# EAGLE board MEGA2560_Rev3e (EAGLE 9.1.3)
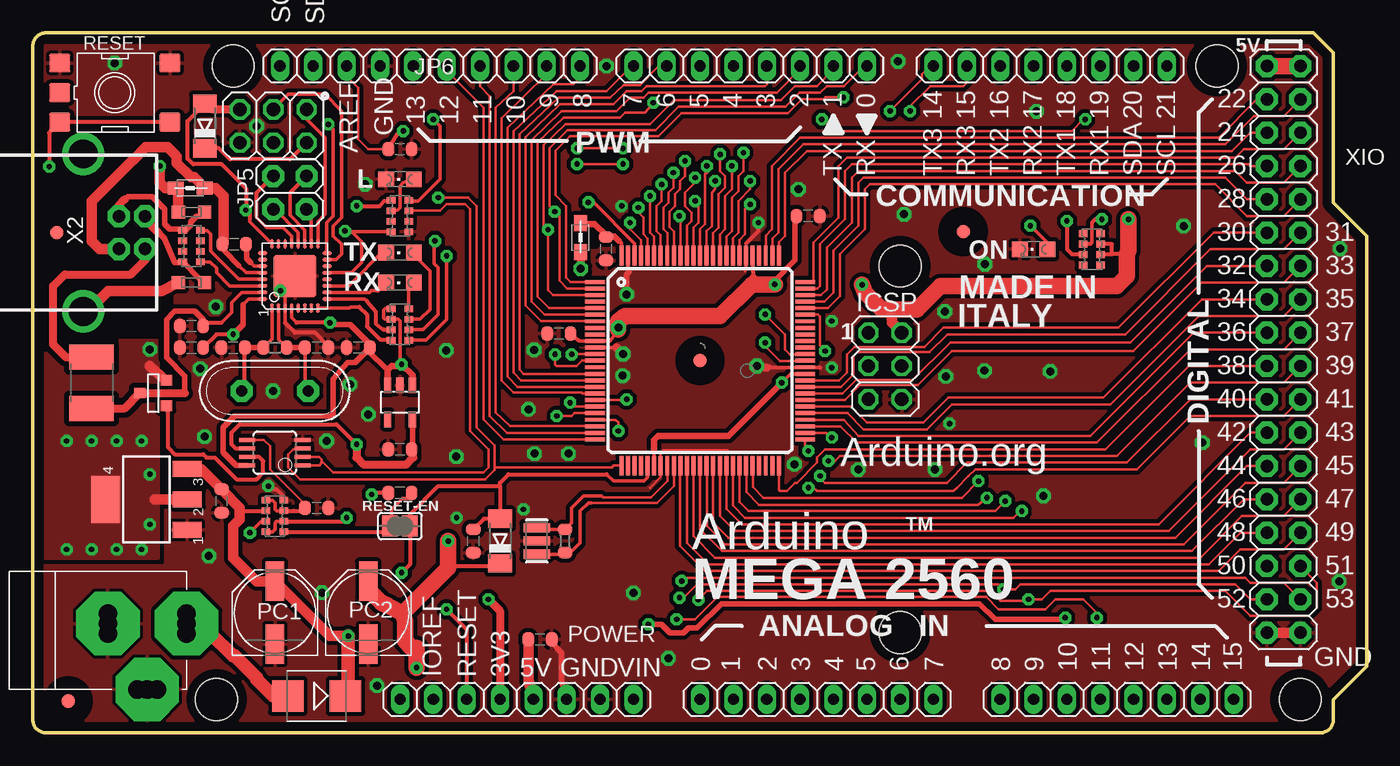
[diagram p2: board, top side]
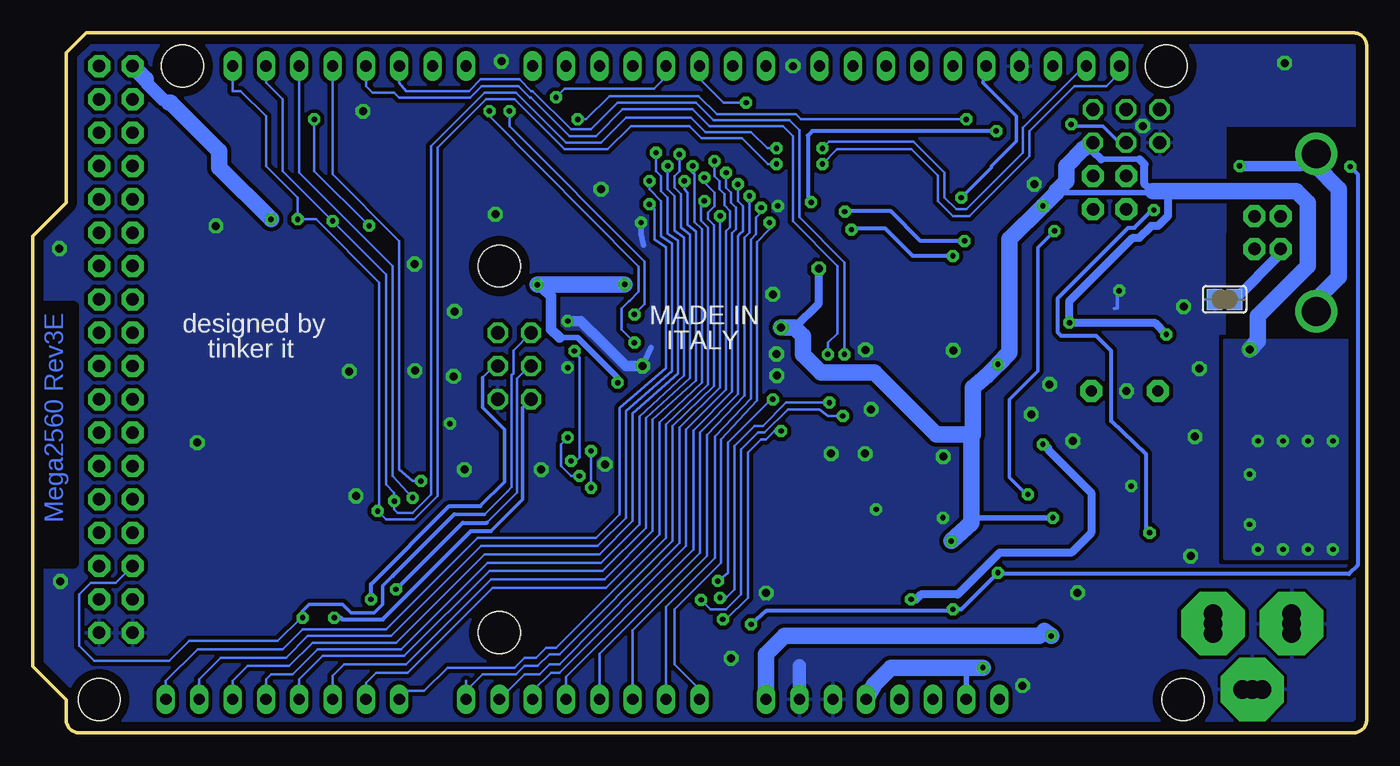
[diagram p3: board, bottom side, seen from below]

Size 101.6 x 53.34 mm. Coordinates in mm from the lower left corner, seen from the top.
Outline: 97.54,53.34 99.06,51.82 99.06,40.39 101.6,37.85 101.6,5.08 99.06,2.54 99.06,1 arc-90 98.06,0 1,0 arc-90 0,1 0,52.34 arc-90 1,53.34 97.54,53.34
Copper layers (1*16): Top 0.035mm / dielectric 1.5mm / Bottom 0.035mm
Design rules "ArduinoMega *": minimum track width 8mil, minimum drill 16mil, track to track 7mil, track to pad 7mil, pad to pad 8mil, via to via 10mil, smd to smd 7mil, copper to edge 27mil, drill to drill 12mil, minimum pad ring 10mil, minimum via ring 10mil, stop-mask expansion 2mil, vias tented up to drill 24mil, thermal gap 10mil
Net classes: 0 default: width 0.203 mm, drill 0.406 mm, clearance 0.203 mm; 1 power: width 0.61 mm, drill 0.406 mm, clearance 0.203 mm; 2 gnd: width 0.305 mm, drill 0.406 mm, clearance 0.203 mm; 3 power usb: width 0.508 mm, drill 0.406 mm, clearance 0.203 mm
Holes 3.2 mm at 96.55,2.55 15.27,50.81 90.2,50.81 14,2.55 66.07,35.57 66.07,7.63
tRestrict: area 42.5,37.2 to 42.9,37.4
bRestrict: 3 lines

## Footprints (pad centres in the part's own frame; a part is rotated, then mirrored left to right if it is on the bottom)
1X08 = drill 0.85 pad 1.422 long: 1 -8.89,0; 2 -6.35,0; 3 -3.81,0; 4 -1.27,0; 5 1.27,0; 6 3.81,0; 7 6.35,0; 8 8.89,0
C0603-ROUND = smd 0.898 x 1.1: 1 -0.889,0; 2 0.889,0
SMB = smd 2.4 x 2.4: A 2.2,0; C -2.2,0
MINIMELF = smd 1.4 x 1.8: A 1.7,0; C -1.7,0
L1812 = smd 1.9 x 3.4: 1 -1.95,0; 2 1.95,0
FIDUCIA-MOUNT = smd 1.016 x 1.016: P$1 0,0
SJ = smd 1.168 x 1.6: 1 -0.762,0; 2 0.762,0
LINEAR_SOT223 = smd 1.219 x 2.235: 1 -2.311,-3.099; 2 0,-3.099; 3 2.311,-3.099 | smd 3.6 x 2.2: 4 0,3.099
TQFP100 = smd 1.5 x 0.3: 1 -8,6; 2 -8,5.5; 3 -8,5; 4 -8,4.5; 5 -8,4; 6 -8,3.5; 7 -8,3; 8 -8,2.5; 9 -8,2; 10 -8,1.5; 11 -8,1; 12 -8,0.5; 13 -8,0; 14 -8,-0.5; 15 -8,-1; 16 -8,-1.5; 17 -8,-2; 18 -8,-2.5; 19 -8,-3; 20 -8,-3.5; 21 -8,-4; 22 -8,-4.5; 23 -8,-5; 24 -8,-5.5; 25 -8,-6; 51 8,-6; 52 8,-5.5; 53 8,-5; 54 8,-4.5; 55 8,-4; 56 8,-3.5; 57 8,-3; 58 8,-2.5; 59 8,-2; 60 8,-1.5; 61 8,-1; 62 8,-0.5; 63 8,0; 64 8,0.5; 65 8,1; 66 8,1.5; 67 8,2; 68 8,2.5; 69 8,3; 70 8,3.5; 71 8,4; 72 8,4.5; 73 8,5; 74 8,5.5; 75 8,6 | smd 0.3 x 1.5: 26 -6,-8; 27 -5.5,-8; 28 -5,-8; 29 -4.5,-8; 30 -4,-8; 31 -3.5,-8; 32 -3,-8; 33 -2.5,-8; 34 -2,-8; 35 -1.5,-8; 36 -1,-8; 37 -0.5,-8; 38 0,-8; 39 0.5,-8; 40 1,-8; 41 1.5,-8; 42 2,-8; 43 2.5,-8; 44 3,-8; 45 3.5,-8; 46 4,-8; 47 4.5,-8; 48 5,-8; 49 5.5,-8; 50 6,-8; 76 6,8; 77 5.5,8; 78 5,8; 79 4.5,8; 80 4,8; 81 3.5,8; 82 3,8; 83 2.5,8; 84 2,8; 85 1.5,8; 86 1,8; 87 0.5,8; 88 0,8; 89 -0.5,8; 90 -1,8; 91 -1.5,8; 92 -2,8; 93 -2.5,8; 94 -3,8; 95 -3.5,8; 96 -4,8; 97 -4.5,8; 98 -5,8; 99 -5.5,8; 100 -6,8
MLF32 = smd 0.7 x 0.28: 1 -2.45,1.75; 2 -2.45,1.25; 3 -2.45,0.75; 4 -2.45,0.25; 5 -2.45,-0.25; 6 -2.45,-0.75; 7 -2.45,-1.25; 8 -2.45,-1.75; 17 2.45,-1.75; 18 2.45,-1.25; 19 2.45,-0.75; 20 2.45,-0.25; 21 2.45,0.25; 22 2.45,0.75; 23 2.45,1.25; 24 2.45,1.75 | smd 0.28 x 0.7: 9 -1.75,-2.45; 10 -1.25,-2.45; 11 -0.75,-2.45; 12 -0.25,-2.45; 13 0.25,-2.45; 14 0.75,-2.45; 15 1.25,-2.45; 16 1.75,-2.45; 25 1.75,2.45; 26 1.25,2.45; 27 0.75,2.45; 28 0.25,2.45; 29 -0.25,2.45; 30 -0.75,2.45; 31 -1.25,2.45; 32 -1.75,2.45 | smd 3.254 x 3.254: 33 0,0
SOT23-DBV = smd 0.55 x 1.2: 1 -0.95,-1.3; 2 0,-1.3; 3 0.95,-1.3; 4 0.95,1.3; 5 -0.95,1.3
MSOP08 = smd 0.3 x 1.2: 1 -0.976,-2.113; 2 -0.326,-2.113; 3 0.324,-2.113; 4 0.974,-2.113; 5 0.974,2.112; 6 0.324,2.112; 7 -0.326,2.112; 8 -0.976,2.112
2X03 = drill 1.016 pad 1.55 octagon: 1 -2.54,-1.27; 2 -2.54,1.27; 3 0,-1.27; 4 0,1.27; 5 2.54,-1.27; 6 2.54,1.27
2X02 = drill 0.95 pad 1.676 octagon: 1 -1.27,-1.27; 2 -1.27,1.27; 3 1.27,-1.27; 4 1.27,1.27
1X10 = drill 0.85 pad 1.422 long: 1 -11.43,0; 2 -8.89,0; 3 -6.35,0; 4 -3.81,0; 5 -1.27,0; 6 1.27,0; 7 3.81,0; 8 6.35,0; 9 8.89,0; 10 11.43,0
CHIPLED_0805 = smd 1.2 x 1.2: A 0,-1.05; C 0,1.05
0805 = smd 1.2 x 1: 1 -1.1,0; 2 1.1,0
PANASONIC_D = smd 3 x 1.4: + 2.4,0; - -2.4,0
R0603-ROUND = smd 0.898 x 1.1: 1 -0.889,0; 2 0.889,0
TS42 = smd 1.6 x 1.4: 1 -4.2,2.25; 2 4.2,2.25; 3 -4.2,-2.25; 4 4.2,-2.25; 5 -4.2,0
CAY16 = smd 0.5 x 0.65: 1 -1.2,-0.675; 2 -0.4,-0.675; 3 0.4,-0.675; 4 1.2,-0.675; 5 1.2,0.675; 6 0.4,0.675; 7 -0.4,0.675; 8 -1.2,0.675
SOT-23 = smd 0.787 x 0.889: 1 0.025,-1.016; 2 -0.94,1.016; 3 0.991,1.016
POWERSUPPLY_DC-21MM = drill 1.4 pad 4.826 octagon: 1 -5.08,-3.353; 2 -0.076,-6.35; 3 -0.076,-0.356 | drill 1.4: 4 -5.08,-4.115; 5 -5.08,-2.591; 6 -0.838,-0.356; 7 0.686,-0.356; 8 -0.838,-6.35; 9 0.686,-6.35
PN61729 = drill 0.95 pad 1.676 octagon: 1 1.25,4.71; 2 -1.25,4.71; 3 -1.25,2.71; 4 1.25,2.71 | drill 2.2: P$1 -6,0; P$2 6,0
2X18 = drill 0.95 pad 1.676 octagon: 1 -21.59,-1.27; 2 -21.59,1.27; 3 -19.05,-1.27; 4 -19.05,1.27; 5 -16.51,-1.27; 6 -16.51,1.27; 7 -13.97,-1.27; 8 -13.97,1.27; 9 -11.43,-1.27; 10 -11.43,1.27; 11 -8.89,-1.27; 12 -8.89,1.27; 13 -6.35,-1.27; 14 -6.35,1.27; 15 -3.81,-1.27; 16 -3.81,1.27; 17 -1.27,-1.27; 18 -1.27,1.27; 19 1.27,-1.27; 20 1.27,1.27; 21 3.81,-1.27; 22 3.81,1.27; 23 6.35,-1.27; 24 6.35,1.27; 25 8.89,-1.27; 26 8.89,1.27; 27 11.43,-1.27; 28 11.43,1.27; 29 13.97,-1.27; 30 13.97,1.27; 31 16.51,-1.27; 32 16.51,1.27; 33 19.05,-1.27; 34 19.05,1.27; 35 21.59,-1.27; 36 21.59,1.27
RESONATOR = smd 0.7 x 2: 1 -1,0; 2 0,0; 3 1,0
QS = drill 0.85 pad 1.676 octagon: 1 -2.54,0; 2 2.54,0
CT/CN0603 = smd 1 x 1: 1 -1,0; 2 1,0

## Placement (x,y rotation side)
ADCH  FH254-108DF08500V  [1X08]  82.58,2.55 0 top
ADCL  FH254-108DF08500V  [1X08]  59.72,2.55 0 top
C1  22p  [C0603-ROUND]  33.55,14.62 270 top
C2  100nF  [C0603-ROUND]  14.38,17.67 270 top
C3  100nF  [C0603-ROUND]  27.97,44.46 0 top
C4  100nF  [C0603-ROUND]  38.63,7.12 0 top
C5  100nF  [C0603-ROUND]  59.06,39.38 0 top
C6  100nF  [C0603-ROUND]  40.07,30.43 180 top
C7  100nF  [C0603-ROUND]  27.97,18.3 0 top
C8  100nF  [C0603-ROUND]  12.09,31 180 top
C9  100nF  [C0603-ROUND]  12.09,29.35 180 top
C10  1uF  [C0603-ROUND]  15.34,37.22 180 top
C11  100nF  [C0603-ROUND]  24.79,29.35 0 top
C12  100nF  [C0603-ROUND]  21.62,17.16 180 top
C13  1uF  [C0603-ROUND]  27.97,21.6 0 top
C14  22p  [C0603-ROUND]  15.27,29.35 180 top
C15  22p  [C0603-ROUND]  21.62,29.35 0 top
C16  100nF  [C0603-ROUND]  43.66,36.88 270 top
COMMUNICATION  FH254-108DF08500V  [1X08]  77.5,50.81 180 top
D1  M7  [SMB]  21.62,2.81 180 top
D2  CD1206-S01575  [MINIMELF]  13.11,46.24 90 top
D3  CD1206-S01575  [MINIMELF]  35.59,14.62 90 top
F1  MF-MSMF050-2 500mA  [L1812]  4.47,26.68 90 top
FD1  FIDUCIALMOUNT  [FIDUCIA-MOUNT]  70.87,38.2 0 top
FD2  FIDUCIALMOUNT  [FIDUCIA-MOUNT]  2.69,2.43 0 top
FD3  FIDUCIALMOUNT  [FIDUCIA-MOUNT]  1.8,38.11 0 top
FD4  FIDUCIALMOUNT  [FIDUCIA-MOUNT]  50.83,28.36 0 top
FRAME2  [FRAME]  not placed on the board
GROUND  [SJ]  10.82,33.03 180 bottom
IC1  1870_LD1117S50CTR  [LINEAR_SOT223]  8.66,17.79 90 top
IC3  ATMEGA2560-15AU  [TQFP100]  50.83,28.36 0 top
IC4  ATMEGA16U2-MU  [MLF32]  19.96,34.81 90 top
IC6  LP2985-33DBVR  [SOT23-DBV]  27.97,25.18 180 top
IC7  LMV358IDGKR  [MSOP08]  18.44,21.35 90 top
ICSP  ICSP  [2X03]  64.92,27.95 270 top
ICSP1  ICSP  [2X03]  18.31,46.24 180 top
JP5  2x2M - NM  [2X02]  19.58,41.16 90 top
JP6  FH254-110DF08500V  [1X10]  30.25,50.81 0 top
L  Yellow  [CHIPLED_0805]  27.97,42.18 90 top
L1  MH2029-300Y  [0805]  11.99,41.52 180 top
L2  10uH  [0805]  41.71,37.74 270 top
ON  Green  [CHIPLED_0805]  76.23,36.84 90 top
PC1  47uF  [PANASONIC_D]  18.44,9.16 90 top
PC2  47uF  [PANASONIC_D]  25.55,9.16 90 top
POWER  FH254-108DF08500V  [1X08]  36.86,2.55 0 top
PWML  FH254-108DF08500V  [1X08]  54.64,50.81 180 top
R1  1M  [R0603-ROUND]  40.54,14.62 90 top
R2  1M  [R0603-ROUND]  18.44,29.35 0 top
RESET  TS42  [TS42]  6.25,48.78 0 top
RESET-EN  [SJ]  27.97,15.76 0 top
RN1  10k  [CAY16]  80.67,36.84 270 top
RN2  22R  [CAY16]  12.09,37.1 90 top
RN3  1K  [CAY16]  27.97,39.38 270 top
RN4  1K  [CAY16]  27.97,31.13 90 top
RN5  10k  [CAY16]  18.44,16.52 90 top
RX  Yellow  [CHIPLED_0805]  27.97,34.3 90 top
T1  PMV48XP  [SOT-23]  9.17,25.92 270 top
TX  Yellow  [CHIPLED_0805]  27.97,36.59 90 top
X1  POWERSUPPLY_DC21MMX  [POWERSUPPLY_DC-21MM]  5.36,8.39 90 top
X2  [PN61729]  3.84,38.11 270 top
XIO  18x2F-H8.5  [2X18]  95.28,29.22 270 top
Y1  CSTCE16M0V53-R0  [RESONATOR]  38.38,14.62 270 top
Y2  16MHz  [QS]  18.44,26.05 180 top
Z1  BRNCG0603MLC-05E  [CT/CN0603]  12.09,34.3 0 top
Z2  BRNCG0603MLC-05E  [CT/CN0603]  12.09,39.69 0 top

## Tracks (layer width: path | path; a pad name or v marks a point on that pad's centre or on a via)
8PB4
  Top 0.254: 20.6,39.89 JP5.1 21.21,39.53 IC4.18
8PB5
  Top 0.254: 19.58,41.16 19.58,39.43 20.71,38.3 IC4.19
  Top 0.305: 19.58,41.16 JP5.3
8PB6
  Top 0.254: IC4.20 20.21,38.12 18.44,39.89 JP5.2
8PB7
  Top 0.254: IC4.21 19.71,37.86 19.08,38.49 17.81,38.49 17.04,39.26 17.04,39.38
  Top 0.305: 17.04,39.38 17.04,41.16 JP5.4
+3V3  (via drill 0.41)
  Top 0.305: IC7.6 15.45,21.67 15.14,21.98 15.14,22.87 15.77,23.51 23.14,23.51 v24.66,21.98
  Top 0.406: 28.92,21.63 IC6.5
  Top 0.61: POWER.4 35.59,9.28 v34.7,10.17 | 28.92,21.63 C13.2 28.98,21.56 28.98,20.97 28.47,20.46 25.17,20.46 24.66,20.97 v24.66,21.98
  Bottom 0.61: v34.7,10.17 34.32,10.17 33.93,10.55 31.14,10.55 27.97,13.73 22.5,13.73 20.98,15.25 20.98,18.3 24.28,21.6 24.28,21.73 v24.66,21.98
+5V  (via drill 0.41, 0.61)
  Top 0.254: IC3.80 54.84,36.31 54.81,36.28 54.84,36.26 54.84,35.42 | 57.68,27.32 57.72,27.36 | v28.09,28.08 28.03,28.21 27.97,28.65 27.97,31.38 27.82,31.53 RN4.6 26.81,31.53 26.73,31.61 26.73,32.21 26.84,32.33 RN4.5 | RN5.8 18.26,15.32 18.44,15.51 18.44,16.01 18.55,16.12 RN5.2 | IC4.32 16.44,33.06 16.03,32.65
  Top 0.279: 57.72,27.36 IC3.61 | v57.05,26.68 57.68,27.32 | 44.48,30.49 43.97,29.86 IC3.10 41.62,29.86 | IC4.4 19.71,31.63 20.09,31.25 | IC3.31 47.33,21.53
  Top 0.305: 54.89,34.68 54.89,35.12 54.84,35.17 54.84,35.42 | 83.34,36.46 82.19,36.46 | v24.66,40.14 26.44,40.14 26.76,40.53 RN3.1 | RN1.6 82.18,36.44 82.19,36.46 | 82.19,36.46 82.19,37.22 82.18,37.24 RN1.7 | 41.62,29.86 C6.1 | C9.1 14,30.37 v15.27,30.37 | RN5.2 23.63,16.12 v23.9,16.4 | v22.63,31.25 20.09,31.25 | D2.C 14.17,44.54 15.01,43.7 19.58,43.7 ICSP1.2 | D3.C 35.03,12.92 34.82,12.71 32.66,12.71 31.7,12.71 31.95,12.92 31.65,13.22
  Top 0.406: 44.57,30.72 44.48,30.49 v44.6,30.87 | v56.52,34.18 56.52,34.4 56.54,34.48 58.06,36.03 58.06,39.28 C5.1 | C11.2 25.55,29.1 27.02,27.64 | C11.2 25.68,29.6 24.16,31.13 22.76,31.13 v22.63,31.25 | C11.2 24.54,28.21 23.99,28.21 22.89,26.98 22.89,24.27 22.63,24.14 15.39,24.14 14.5,23.25 14.5,21.35 15.49,20.36 16.34,20.36 IC7.8 | 16.03,32.65 16.03,31.13 v15.27,30.37
  Top 0.508: v57.05,26.68 52.98,22.62 47.63,22.62 47.32,22.31 47.32,21.53 47.33,21.53 | 26.99,26.68 IC6.3 27.02,27.64 27.33,27.95 27.97,27.95 | IC6.1 28.92,27.26 v28.09,28.08
  Top 0.61: v28.09,28.08 27.97,27.95 | 54.89,34.68 54.89,34.3 55.02,34.18 | L2.2 41.71,35.34 v41.73,35.37
  Top 0.813: 9.3,17.79 IC1.2 | C4.1 37.74,3.95 POWER.5 | 83.34,34.81 83.34,34.94 | 65.43,32.27 65.43,31.25 ICSP.2 | T1.2 10.13,26.86 8.92,27.95
  Top 1.27: XIO.1 XIO.2 | v63.17,34.15 63.4,33.54 64.67,32.27 65.43,32.27 67.34,32.27 69.11,34.05 82.58,34.05 83.34,34.81 | 83.34,34.94 83.34,36.46 83.46,36.72 v83.46,39.13 | 44.57,30.72 44.57,31.35 45.11,31.76 52.35,31.76 54.76,34.18 55.02,34.18 v56.52,34.18 | v31.65,14.62 31.65,13.22 31.65,12.59 28.16,9.09 | v29.24,4.97 29.24,6.49 28.85,6.49 28.35,7 28.35,8.52 28.16,9.09 | PC2.+ 25.55,10.93 26.57,9.92 27.08,9.66 28.16,9.09
  Bottom 0.406: v44.6,30.87 44.6,30.75 | 61.49,30.11 60.1,30.11 57.05,27.06 v57.05,26.68 | 23.52,41.16 16.79,41.16 16.66,41.29 16.28,41.29 | 17.3,43.7 20.22,43.7 | v23.9,16.4 30.12,16.4 | POWER.2 30.51,4.76 30.71,4.97
  Bottom 0.61: 63.14,34.18 v63.17,34.15 | 23.65,41.29 23.52,41.16 | 16.28,41.29 16.92,41.8 16.92,43.32 17.3,43.7 | 20.22,43.7 20.85,44.34 ICSP1.2 | v15.27,30.37 16.15,31.25 v22.63,31.25 22.63,32.91 17.81,37.73 17.3,37.73 16.41,38.62 15.9,38.62 15.14,39.38 15.14,41.29 | 43.59,30.87 41.73,32.73 v41.73,35.37
  Bottom 0.813: 61.49,30.11 62.13,30.75 62.13,33.29 v63.17,34.15
  Bottom 1.016: 91.21,48.02 91.72,48.27 92.86,49.42 92.99,49.8
  Bottom 1.27: v29.24,4.97 30.71,4.97 36.22,4.97 37.49,3.7 POWER.5 | v56.52,34.18 63.14,34.18 | v44.6,30.87 43.59,30.87 42.95,30.24 42.95,28.84 41.55,27.44 37.49,27.44 32.79,22.75 30.12,22.75 | ICSP1.2 20.98,44.84 21.62,44.46 22.89,43.19 22.89,42.05 23.65,41.29 23.65,41.16 v24.66,40.14 27.2,37.6 27.2,28.97 v28.09,28.08 28.98,27.19 30,26.3 30,22.75 30.12,22.75 | 30.12,22.75 30.12,16.4 30.12,16.01 v31.65,14.62 | v83.46,39.13 87.4,43.07 87.4,44.34 91.08,48.02 91.21,48.02 | v8.92,29.22 8.28,29.86 8.28,31.76 4.47,35.57 4.47,40.4 5.36,41.29 15.14,41.29 16.28,41.29 | 92.99,49.8 XIO.1
  other vias: 6.38,22.24 4.47,22.24 8.28,22.24 2.57,22.24 8.92,19.7 2.57,13.98 6.38,13.98 4.47,13.98 8.92,15.89 8.28,13.98
  pour Top (isolate 0.406, no thermals): 9.55,13.35 9.55,29.86 0.66,29.86 0.66,13.35
  pour Bottom: 1.5,13.35 1.5,29.86 10.82,29.86 10.82,13.35
ADC0  (via drill 0.41)
  Top 0.203: IC3.97 46.33,37.53 45.49,38.37 v45.49,38.87
  Bottom 0.203: ADCL.1 50.83,3.31 52.73,5.22 52.73,9.41 49.17,12.97 49.17,22.36 46.43,25.34 46.43,37.4 45.49,38.37 v45.49,38.87
ADC1  (via drill 0.41)
  Top 0.203: IC3.96 46.83,37.67 46.51,37.99 46.51,39.26 46.13,39.64 v46.13,40.02
  Bottom 0.203: ADCL.2 53.37,9.61 49.66,13.32 49.66,22.57 46.91,25.46 46.91,37.58 46.51,37.99 46.51,39.26 46.13,39.64 v46.13,40.02
ADC2  (via drill 0.41)
  Top 0.203: v47.02,40.91 47.02,38.11 47.32,37.81 IC3.95 47.29,36.36
  Bottom 0.203: ADCL.3 55.91,7.81 50.24,13.47 50.24,22.69 47.4,25.69 47.4,37.73 47.02,38.11 v47.02,40.91
ADC3  (via drill 0.41)
  Top 0.203: IC3.94 47.83,37.94 47.52,38.24 47.52,40.14 47.9,40.53 v47.9,41.8
  Bottom 0.203: ADCL.4 58.45,2.76 58.55,2.86 58.55,3.06 58.45,3.16 58.45,6.03 50.77,13.7 50.77,22.87 47.88,25.82 47.88,37.86 47.78,37.99 47.52,38.24 47.52,40.14 47.9,40.53 v47.9,41.8
ADC4  (via drill 0.41)
  Top 0.203: IC3.93 48.33,38.07 48.03,38.37 48.03,40.02 48.41,40.4 48.41,41.16 48.79,41.54 v48.79,42.68
  Bottom 0.203: 60.99,2.45 ADCL.5 60.99,4.28 51.28,13.98 51.28,23.02 48.34,26.02 48.34,38.06 48.03,38.37 48.03,40.02 48.41,40.4 48.41,41.16 48.79,41.54 v48.79,42.68
ADC5  (via drill 0.41)
  Top 0.203: IC3.92 48.83,38.21 48.49,38.54 48.49,39.71 48.92,40.14 48.92,41.03 49.3,41.41 49.3,42.05 49.68,42.43 v49.68,43.57
  Bottom 0.203: v49.68,43.57 49.68,42.43 49.3,42.05 49.3,41.41 48.92,41.03 48.92,40.2 48.49,39.76 48.49,38.54 48.79,38.24 48.79,26.17 51.84,23.13 51.84,14.24 61.49,4.58 62.13,4.58 63.53,3.19 ADCL.6
ADC6  (via drill 0.41)
  Top 0.203: IC3.91 49.33,39.36 v49.25,39.38
  Bottom 0.203: v49.25,39.38 49.25,26.3 52.35,23.25 52.35,14.49 61.49,5.22 62.26,5.22 63.02,4.46 64.16,4.46 ADCL.7
ADC7  (via drill 0.41)
  Top 0.203: IC3.90 49.83,38.64 50.19,39 50.19,39.64 49.68,40.14 49.68,41.16 50.44,41.92 v50.44,42.3
  Bottom 0.203: v50.44,42.3 50.44,41.92 49.68,41.16 49.68,40.14 50.19,39.64 50.19,39.15 49.71,38.67 49.71,26.43 52.86,23.38 52.86,14.62 61.49,5.98 62.26,5.98 63.14,5.09 64.16,5.09 64.8,4.46 67.34,4.46 68.61,3.19 | 68.61,3.19 ADCL.8 | 68.61,3.19 68.61,3.95
ADC8  (via drill 0.41)
  Top 0.203: IC3.89 50.33,38.5 50.7,38.87 50.7,40.27 v50.44,40.53
  Bottom 0.203: v50.44,40.53 50.7,40.27 50.7,39.03 50.17,38.49 50.17,26.56 53.37,23.51 53.37,14.87 61.75,6.49 62.51,6.49 63.27,5.73 64.16,5.73 64.92,4.97 70,4.97 71.78,3.19 73.69,3.19 ADCH.1
ADC9  (via drill 0.41)
  Top 0.203: IC3.88 50.83,38.37 51.21,38.75 51.21,42.56 51.33,42.68 v51.33,43.19
  Bottom 0.203: v51.33,43.19 51.33,42.68 51.21,42.56 51.21,38.9 50.62,38.37 50.62,26.68 53.87,23.63 53.87,15.13 57.94,11.06 66.57,11.06 73.05,4.58 75.46,4.58 76.23,3.82 ADCH.2
ADC10  (via drill 0.41)
  Top 0.203: IC3.87 51.33,38.23 51.71,38.62 51.71,41.16 51.97,41.41 v51.97,42.05
  Bottom 0.203: v51.97,42.05 51.97,41.41 51.71,41.16 51.71,38.72 51.08,38.19 51.08,26.86 54.38,23.86 54.38,15.38 58.06,11.7 66.7,11.7 73.18,5.22 77.88,5.22 78.77,4.33 ADCH.3
ADC11  (via drill 0.41)
  Top 0.203: IC3.86 51.83,38.1 52.22,38.49 52.22,41.03 52.73,41.54 52.73,42.43 52.35,42.81 v52.35,44.08
  Bottom 0.203: v52.35,44.08 52.35,42.81 52.73,42.43 52.73,41.54 52.22,41.03 52.22,38.49 51.54,37.96 51.54,27.04 54.89,23.99 54.89,15.63 58.19,12.33 66.83,12.33 73.3,5.85 79.53,5.85 81.31,4.08 ADCH.4
ADC12  (via drill 0.41)
  Top 0.203: IC3.85 52.33,37.96 52.73,38.37 52.73,40.91 53.24,41.41 v53.24,43.19
  Bottom 0.203: v53.24,43.19 53.24,41.41 52.73,40.91 52.73,38.26 51.99,37.73 51.99,27.22 55.4,24.12 55.4,15.89 58.32,12.97 66.95,12.97 73.56,6.36 79.91,6.36 81.81,4.46 83.46,4.46 83.85,4.08 ADCH.5
ADC13  (via drill 0.41)
  Top 0.203: IC3.84 52.83,37.83 53.24,38.24 53.24,40.78 53.75,41.29 53.75,42.43 54.13,42.81 v54.13,44.21
  Bottom 0.203: v54.13,44.21 54.13,42.81 53.75,42.43 53.75,41.29 53.24,40.78 53.24,38.04 52.45,37.5 52.45,27.39 55.91,24.35 55.91,16.14 58.45,13.6 67.21,13.6 73.94,6.87 80.29,6.87 82.07,5.09 85.24,5.09 86.39,3.95 ADCH.6
ADC14  (via drill 0.41)
  Top 0.203: IC3.83 53.33,37.69 53.75,38.11 53.75,40.53 54.64,41.41 v54.64,42.05
  Bottom 0.203: v54.64,42.05 54.64,41.41 53.75,40.53 53.75,37.86 52.91,37.27 52.91,27.57 56.41,24.52 56.41,16.4 58.57,14.24 67.46,14.24 74.32,7.38 80.67,7.38 82.32,5.73 87.27,5.73 88.93,4.08 ADCH.7
ADC15  (via drill 0.41)
  Top 0.203: IC3.82 53.83,37.56 54.25,37.99 54.25,39.89 v54.64,40.27
  Bottom 0.203: v54.64,40.27 54.25,39.89 54.25,37.58 53.37,36.99 53.37,27.8 56.92,24.75 56.92,16.65 58.7,14.87 67.72,14.87 74.7,7.89 81.05,7.89 82.58,6.36 89.05,6.36 91.47,3.95 ADCH.8
AREF  (via drill 0.41)
  Top 0.203: C3.1 25.55,44.46 24.79,45.22 24.79,49.16 23.9,50.05 JP6.3
  Top 0.254: IC3.98 45.83,37.3 42.7,40.42 v42.32,40.42
  Top 0.305: v28.22,45.86 27.75,45.61 C3.1
  Bottom 0.305: v42.32,40.42 42.57,40.7 42.57,45.5 42.21,45.86 v28.22,45.86
AVCC
  Top 0.279: IC3.100 44.83,37.31
  Top 0.305: 44.83,37.31 44.63,37.5
  Top 0.508: 44.63,37.5 44.32,37.81 43.7,37.81 C16.1 43.66,37.91 42.8,38.77 41.94,38.77 L2.1
CMP
  Top 0.203: C12.2 20.73,17.41 18.06,20.08 18.06,21.86 17.59,22.32 IC7.5
  Top 0.254: 19.1,16.9 18.57,16.9 18.44,17.03 18.44,17.54 18.26,17.72 RN5.5
  Top 0.305: 19.1,16.9 RN5.3 | RN5.3 19.9,16.92 | C12.2 20.49,16.92 RN5.3
D+
  Top 0.406: 7.01,40.65 7.23,40.87 9.08,40.87 10.06,39.89 10.06,38.75 10.44,38.37 11.35,38.37 RN2.5 11.64,38.3 12.04,38.7 12.04,38.93 12.47,39.36 12.76,39.36 Z2.2 12.96,39.51
  Top 0.61: X2.3 6.55,40.19 7.01,40.65
D-
  Top 0.406: 9.55,38.11 9.59,38.11 10.06,37.64 10.06,37.6 10.82,35.83 11.35,35.83 RN2.8 12.76,34.56 Z1.2
  Top 0.61: X2.2 8.55,39.11 9.55,38.11
DTR  (via drill 0.41)
  Top 0.254: 24.28,38.18 23.83,38.18 v23.77,38.24 | 24.28,38.18 RN3.4 | IC4.13 24.28,35.06 25.04,35.83 25.04,37.42 24.28,38.18
  Top 0.305: C7.1 26.06,18.3 v25.81,18.17
  Bottom 0.254: v25.81,18.17 25.93,18.17 27.2,19.44 27.2,25.41 25.04,27.57 25.04,36.97 v23.77,38.24
GATE_CMD
  Top 0.305: T1.3 10.31,24.8 10.31,21.73 10.82,21.22 12.98,21.22 13.23,20.97 13.87,20.97 15.52,19.32 17.04,19.32 17.55,19.82 17.55,20.71 17.24,21.02 IC7.7
  Top 0.406: T1.3 10.19,24.65
GND  (via drill 0.41, 0.61)
  Top 0.203: 54.25,35.19 54.33,35.26 IC3.81 54.36,36.36 | 54.33,37.29 54.33,36.39 54.36,36.36 | IC3.32 47.83,21.25 48.06,21.53 52.91,21.53 | IC3.32 | IC3.32 47.83,19.49 47.02,18.68 | 54.36,36.36 54.28,36.39
  Top 0.279: 45.33,35.22 IC3.99 | 58.85,27.85 58.84,27.86 IC3.62 58.83,27.85 | 56.11,27.85 58.83,27.85 | 58.83,27.85 59.94,27.85 | 19.21,31.24 IC4.3 | 19.21,33.34 19.21,33.37 19.22,33.38 19.22,32.31 | 42.88,29.36 | 42.88,29.36 44.35,29.36 | IC3.11 42.88,29.36
  Top 0.305: IC1.1 11.84,15.51 | 45.42,35.12 45.33,35.22 | 44.42,29.37 44.35,29.36 44.37,29.37 44.45,29.37 | 56.11,27.85 56.08,27.88 | 54.33,37.29 55.27,38.24 v55.27,38.87 | 59.94,27.85 59.97,27.83 | v18.85,33.69 19.26,33.69 | C15.2 22.5,29.48 21.49,30.49 19.96,30.49 19.21,31.24 | IC4.33 19.96,33.34 v18.85,33.69 | v18.85,33.69 19.21,33.33 | 19.21,33.34 v18.85,33.69 | RN5.4 19.12,18.01 18.57,18.55 18.19,18.55 v17.93,18.81
  Top 0.406: C4.2 39.9,6.49 40.28,6.11 40.28,3.95 POWER.6 | 56.08,27.88 56.03,27.83 v55.14,27.95 | v45.24,33.41 45.24,34.94 45.42,35.12
  Top 0.61: v55.14,27.95 55.91,27.83 | 44.45,29.37 v44.96,28.87
  Top 0.813: XIO.35 XIO.36
  Bottom 0.279: 19.21,32.34 19.23,32.34 18.97,32.37 18.97,33.39
  Bottom 0.305: GROUND.2 10.19,33.03
  Bottom 0.406: v44.96,28.87 45.11,29.1 | v55.27,38.87 55.27,37.99 55.07,37.17 | v55.14,27.95 54.51,29.35
  Bottom 0.813: v60.86,31.38 59.89,31.38 59,30.49 58.95,30.49 56.41,27.95 v55.14,27.95 | 93.75,7.89 XIO.35
  Bottom 1.016: POWER.7 43.21,5.09
  other vias: 68.72,20.06 38.2,21.27 31.5,29.15 38.18,29.19 87.66,38.62 89.08,22.11 72.52,35.73 22.02,10.68 13.41,13.47 32.28,16.4 40.79,21.27 17.04,46.24 25.55,24.27 58.32,41.41 76.45,47.36 44.86,40.14 44.93,27.22 48.41,5.68 26.21,3.59 13.08,22.57 24.16,26.56 25.32,41.8 60.86,27.83 58.01,20.46 12.75,27.75 37.74,24.65 77.5,27.55 76.99,18.05 99.58,36.89 69.82,23.56 72.49,27.6 18.29,26.05 69.48,32.11 62.87,20.06 99.5,11.54 65.91,51.17 43.7,50.81 13.94,32.47 66.37,39.51 69.55,27.17 37.36,17.03 32.26,21.04 22.38,22.24 45.75,10.66 6.25,51.04
  pour Top (isolate 0.305, rank 2): 0.36,52.72 101.63,52.72 101.63,0.65 0.66,0.65 0.66,29.86 10.82,29.86 10.77,45.91 0.3,45.91
  pour Bottom (isolate 0.305, rank 2): 0.66,52.72 101.63,52.72 102.26,52.08 102.26,0.65 1.3,0.65 0.66,1.28 0.66,29.86 10.82,29.86 10.77,46.27 0.61,46.27
L13
  Top 0.203: RN3.7 31.03,39.78 31.52,40.27 32.92,40.27 33.3,39.89 33.3,23 34.7,21.6 34.7,20.21 34.32,19.82 22.89,19.82 22,20.71 | IC7.2 21.81,21.02 22,20.84 22,20.71 | IC7.1 21.83,20.37 22,20.59 22,20.71
M8RXD
  Top 0.254: 27.27,30.75 RN4.7 | IC4.9 25.27,33.06 25.43,32.91
  Top 0.305: 27.27,30.75 26.7,30.75 26.11,31.2 26.11,32.09 25.43,32.91
M8TXD
  Top 0.254: 24.86,32.46 24.22,32.46 24.12,32.36 IC4.8
  Top 0.305: 24.86,32.46 25.45,31.86 25.45,30.97 26.44,29.98 27.23,29.98 RN4.8
MISO2
  Top 0.254: IC4.17 21.71,38.97 22.25,39.51 22.25,45.35 20.85,46.75 ICSP1.1
MOSI2  (via drill 0.41)
  Top 0.254: v22.5,46.37 22.89,45.99 22.89,39.38 22.38,38.87 22.38,36.72 22.41,36.63 IC4.16
  Bottom 0.254: ICSP1.4 18.82,44.97 20.09,46.24 22.25,46.24 22.38,46.37 v22.5,46.37
N$2
  Top 0.254: RN3.2 27.78,39.83 27.97,40.02 27.97,41.67 28.22,41.92 L.A
N$3  (via drill 0.41)
  Top 0.203: 77.24,37.1 ON.A | v80.16,46.75 80.04,46.75 79.15,45.86 60.99,45.86 v60.1,46.75
  Top 0.254: v30.51,46.75 31.01,46.24 31.01,42.18 29.36,40.53 28.91,40.53 RN3.8 | 77.24,37.1 77.24,37.38 v75.99,38.64
  Bottom 0.203: v75.99,38.64 80.16,42.81 v80.16,46.75 | v60.1,46.75 59.46,46.75 57.68,48.53 50.88,48.53 49.5,47.15 43.48,47.15 43.08,46.75 v30.51,46.75
N$54
  Top 0.254: RN4.4 28.64,33.83 RX.A
N$55
  Top 0.254: RN4.3 29.51,31.53 30.25,32.27 30.25,35.19 29.02,36.43 TX.A
PA0
  Top 0.203: IC3.78 55.83,37.91 56.29,38.37 56.29,43.19 58.45,45.35 90.32,45.35 93.24,48.27 XIO.3
PA1
  Top 0.203: IC3.77 56.33,37.64 56.79,38.11 56.79,42.94 58.7,44.84 90.83,44.84 92.99,47 95.28,47 XIO.4
PA2
  Top 0.203: XIO.5 92.74,45.73 91.34,44.34 58.95,44.34 57.3,42.68 57.3,37.86 56.83,37.38 IC3.76
PA3
  Top 0.203: XIO.6 95.28,44.46 92.23,44.46 91.59,43.83 62,43.83 61.37,43.19 61.37,39.27 59.46,37.37 59.46,34.53 59.44,34.36 IC3.75
PA4
  Top 0.203: IC3.74 59.78,33.86 59.97,34.05 59.97,37.24 61.87,39.14 61.87,42.81 62.38,43.32 92.61,43.32 92.74,43.19 XIO.7
PA5
  Top 0.203: IC3.73 60.04,33.36 60.48,33.79 60.48,36.99 62.38,38.89 62.38,42.3 62.89,42.81 91.59,42.81 92.48,41.92 95.28,41.92 XIO.8
PA6
  Top 0.203: IC3.72 60.3,32.86 60.99,33.54 60.99,36.73 62.89,38.64 62.89,41.92 63.27,42.3 90.83,42.3 92.48,40.65 XIO.9
PA7
  Top 0.203: IC3.71 60.57,32.36 61.49,33.29 61.49,36.48 63.4,38.38 63.4,41.41 63.78,41.8 90.07,41.8 92.48,39.38 95.28,39.38 XIO.10
PB0  (via drill 0.41)
  Top 0.203: IC3.19 45.42,25.36 v45.24,25.41 | v49.43,11.57 49.56,11.57 49.81,11.82 92.35,11.82 92.74,11.44 95.28,11.44 XIO.34
  Bottom 0.203: v45.24,25.41 45.36,25.41 48.67,22.11 48.67,12.2 v49.43,11.57
PB1  (via drill 0.41)
  Top 0.203: IC3.20 41.22,24.86 v40.92,25.16 | XIO.33 92.74,10.17 91.59,11.32 75.21,11.32 74.83,10.93 v73.94,10.93 73.56,11.32 50.57,11.32 49.56,10.3 v49.26,10.3
  Bottom 0.203: v40.92,25.16 44.22,25.16 46,23.38 46.63,23.38 48.16,21.86 48.16,10.93 48.79,10.3 v49.26,10.3 | 63.78,27.95 64.72,27.01 64.72,18.32 67.03,16.01
  Bottom 0.254: 63.78,27.95 ICSP.3
  Bottom 0.305: 67.03,16.01 68.86,16.01 v73.94,10.93
PB2  (via drill 0.41)
  Top 0.203: IC3.21 41.26,24.36 41.05,24.14 v39.9,24.14 | XIO.32 97.82,11.44 97.82,9.54 97.18,8.9 92.74,8.9 90.83,10.81 77.5,10.81 76.86,10.17 v75.84,10.17 75.72,10.05 73.69,10.05 72.92,10.81 51.37,10.81 v50.7,10.14
  Bottom 0.203: v39.9,24.14 41.05,24.14 41.68,24.65 44.09,24.65 45.87,22.87 46.38,22.87 47.65,21.6 47.65,10.55 48.79,9.41 49.97,9.41 v50.7,10.14 | ICSP.4 66.45,27.95 67.34,27.06
  Bottom 0.254: 67.34,27.06 67.34,24.78 65.68,23.13 65.68,19.12 67.52,17.28
  Bottom 0.305: 67.52,17.28 69.88,17.28 75.84,11.32 v75.84,10.17
PB3  (via drill 0.41)
  Top 0.203: IC3.22 44.38,23.86 44.6,23.63 v44.6,23 | v81.05,8.78 81.05,9.16 80.04,10.17 77.88,10.17 77.11,9.41 73.56,9.41 72.62,10.35 52.15,10.35 50.44,8.65 v49.05,8.65
  Bottom 0.203: v81.05,8.78 81.18,8.78 82.96,7 89.69,7 91.21,5.47 96.93,5.47 98.07,6.62 98.07,10.55 97.18,11.44 95.28,11.44 XIO.31 | v44.6,23 45.11,23 45.75,22.36 46.13,22.36 47.14,21.35 47.14,10.3 48.79,8.65 v49.05,8.65 | ICSP.1 65,29.15 65,27.39 65.13,27.27 65.13,18.73 65.46,18.4 67.21,16.65
  Bottom 0.254: v81.05,8.78 81.05,9.28 80.54,9.79 78,9.79 77.37,9.16 75.59,9.16 74.96,9.79 74.96,11.19 74.19,11.95 | 69.49,16.65 67.21,16.65
  Bottom 0.305: 74.19,11.95 69.49,16.65
PB4
  Top 0.203: IC3.23 42.93,23.36 42.95,23.38 36.35,23.38 35.23,24.4 35.23,47.64 36.6,48.91 JP6.8
PB5
  Top 0.203: IC3.24 36.11,22.86 34.77,24.14 34.77,48.53 34.06,49.29 JP6.7
PB6
  Top 0.203: IC3.25 42.95,22.36 35.84,22.36 34.32,23.89 34.32,47.64 31.78,50.18 JP6.6
PB7  (via drill 0.41)
  Top 0.203: 35.18,20.23 37.62,20.23 | 37.62,20.23 44.12,20.23 44.25,20.36 IC3.26 | v30.89,40.78 33.17,40.78 33.81,40.14 33.81,23.25 35.18,21.88 35.18,20.23 | 37.62,20.23 37.59,20.21 | IC7.3 20.48,21.6 19.84,21.6 19.46,21.22 19.46,20.21 20.35,19.32 34.44,19.32 35.18,20.05 35.18,20.23
  Bottom 0.254: JP6.5 29.24,49.54 26.7,47 26.7,45.1 28.6,43.19 28.6,43.07 v30.89,40.78
PC0
  Top 0.203: IC3.53 61.52,23.36 62.76,22.11 81.05,22.11 88.16,29.22 95.28,29.22 XIO.18
PC1
  Top 0.203: IC3.54 61.78,23.86 62.89,22.62 80.54,22.62 88.42,30.49 XIO.17
PC2
  Top 0.203: IC3.55 62.04,24.36 63.27,23.13 68.1,23.13 70,25.03 82.07,25.03 88.8,31.76 95.28,31.76 XIO.16
PC3
  Top 0.203: IC3.56 62.3,24.86 63.53,23.63 67.84,23.63 69.75,25.54 81.56,25.54 89.05,33.03 XIO.15
PC4
  Top 0.203: IC3.57 61.87,25.36 63.02,26.49 67.41,26.49 70,29.1 83.85,29.1 89.05,34.3 95.28,34.3 XIO.14
PC5
  Top 0.203: IC3.58 61.69,25.86 62.69,26.87 67.01,26.87 69.88,29.73 83.59,29.73 89.43,35.57 XIO.13
PC6
  Top 0.203: IC3.59 61.55,26.36 62.51,27.32 62.51,28.71 62.81,29.03 68.3,29.03 69.65,30.37 83.21,30.37 89.69,36.84 95.28,36.84 XIO.12
PC7
  Top 0.203: IC3.60 61.42,26.86 62,27.44 62,28.84 62.59,29.41 67.89,29.41 69.34,30.87 82.7,30.87 89.94,38.11 XIO.11
PD7
  Top 0.203: XIO.19 88.04,27.95 81.69,21.6 60.33,21.6 60.33,21.58 59.72,20.97 59.72,20.59 58.19,19.06 58.06,19.06 57.43,18.43 56.92,18.43 56.83,18.52 IC3.50
PE0  (via drill 0.41)
  Top 0.203: PWML.1 63.32,50.81 61.8,49.29 60.48,49.29 59.97,48.78 58.39,48.78 57.33,47.71 49.2,47.71 47.42,45.94 40.72,45.94 39.34,44.56 39.34,40.12 v39.75,39.71 39.75,39.69 39.8,39.69 40.11,39.38 40.11,34.45 40.7,33.86 IC3.2
  Top 0.254: v30.63,37.48 30.56,37.41 30.56,35.76 30.89,35.45 30.89,31.89 29.74,30.75 28.66,30.75 RN4.2
  Bottom 0.305: v30.63,37.48 33.99,37.48 36.25,39.74 39.73,39.74 v39.75,39.71
PE1  (via drill 0.41)
  Top 0.203: IC3.3 39.63,33.36 39.24,33.74 v39.24,38.34 38.89,38.7 38.89,44.77 40.56,46.39 47.02,46.39 48.84,48.22 56.97,48.22 58.04,49.29 59.72,49.29 60.99,50.56 PWML.2
  Top 0.254: RN4.1 29.94,29.93 31.52,31.51 v31.52,36.33
  Bottom 0.305: v31.52,36.33 34.57,36.33 36.65,38.42 39.17,38.42 v39.24,38.34
PE3  (via drill 0.41)
  Top 0.203: IC3.5 39.31,32.36 38.43,33.24 38.43,45 40.41,46.88 44.73,46.88 45.11,47.26 46.63,47.26 v47.27,48.02
  Bottom 0.203: v47.27,48.02 49,48.02 50.83,49.85 PWML.6
PE4
  Top 0.203: IC3.6 38.99,31.86 37.97,32.88 37.97,45.17 40.28,47.38 44.48,47.38 45.49,48.4 46.51,48.4 46.89,48.78 56.67,48.78 58.45,50.56 PWML.3
PE5
  Top 0.203: IC3.7 42.8,31.36 42.57,31.38 38.71,31.38 37.52,32.58 37.52,45.4 40.16,47.89 44.22,47.89 45.24,48.91 46.38,48.91 46.76,49.29 55.78,49.29 55.91,49.42 PWML.4
PG0  (via drill 0.41)
  Top 0.203: IC3.51 58.83,21.86 v59.08,21.48 | XIO.22 95.28,24.14 88.16,24.14 84.1,20.08 71.78,20.08 71.27,19.57 70.38,18.68 70.13,18.43 59.72,18.43 59.46,18.68 v59.08,18.68
  Bottom 0.203: v59.08,18.68 v59.08,21.48
PG1  (via drill 0.41)
  Top 0.203: IC3.52 60.46,22.86 v60.86,22.49 | XIO.21 88.16,25.41 83.34,20.59 71.15,20.59 69.62,19.06 60.35,19.06 59.97,19.44 v59.97,19.57
  Bottom 0.203: v59.97,19.57 60.6,19.57 61.37,20.33 61.37,21.98 v60.86,22.49
PG2  (via drill 0.41)
  Top 0.203: IC3.70 59.82,31.86 59.94,31.74 59.94,29.5 v60.35,29.1 | v60.6,20.71 61.11,20.71 61.49,21.09 82.58,21.09 88.16,26.68 95.28,26.68 XIO.20
  Bottom 0.203: v60.6,20.71 60.22,20.71 59.97,20.97 59.97,28.59 v60.35,29.1
PG5  (via drill 0.41)
  Top 0.203: v61.75,48.42 60.38,48.42 60.22,48.27 58.6,48.27 57.53,47.21 49.4,47.21 47.68,45.48 40.92,45.48 39.8,44.36 39.8,40.96 40.61,40.14 40.61,34.71 40.97,34.35 IC3.1
  Bottom 0.203: PWML.5 53.24,50.81 53.24,50.08 53.37,49.95 53.42,49.95 54.28,49.09 61.09,49.09 v61.75,48.42
PH3
  Top 0.203: IC3.15 37.4,27.36 37.06,27.7 37.06,45.63 40.03,48.4 43.97,48.4 44.98,49.36 46.25,49.36 47.65,50.81 PWML.7
PH4
  Top 0.203: IC3.16 37.19,26.86 36.6,27.44 36.6,45.86 39.9,48.91 43.71,48.91 45.62,50.81 PWML.8
PH5
  Top 0.203: IC3.17 36.93,26.36 36.14,27.14 36.14,46.11 39.65,49.42 41.17,49.42 41.68,49.92 JP6.10
PH6
  Top 0.203: IC3.18 41.86,25.86 41.8,25.92 36.6,25.92 35.69,26.83 35.69,46.82 39.14,50.18 JP6.9
PL0
  Top 0.203: 49.3,20.31 49.3,14.24 51.21,12.33 90.32,12.33 91.97,13.98 95.28,13.98 XIO.30
  Top 0.254: IC3.35 49.33,20.33 49.3,20.31
PL1
  Top 0.203: IC3.36 49.83,14.47 51.46,12.84 89.56,12.84 91.97,15.25 XIO.29
PL2
  Top 0.203: XIO.28 95.28,16.52 92.1,16.52 88.93,13.35 51.97,13.35 50.32,15 50.32,20.31 50.33,20.32 IC3.37
  Top 0.254: IC3.37
PL3
  Top 0.203: IC3.38 50.83,15.51 52.48,13.86 88.29,13.86 92.23,17.79 XIO.27
PL4
  Top 0.203: XIO.26 95.28,19.06 92.35,19.06 87.66,14.36 52.73,14.36 51.33,15.76 51.33,20.23 51.33,20.24 51.33,20.29
  Top 0.254: 51.33,20.29 IC3.39
PL5
  Top 0.203: IC3.40 51.83,16.03 52.98,14.87 87.02,14.87 92.48,20.33 XIO.25
PL6
  Top 0.203: XIO.24 95.28,21.6 92.74,21.6 86.51,15.38 53.49,15.38 52.35,16.52 52.35,20.33 IC3.41
  Top 0.254: 52.33,20.33 IC3.41
PL7
  Top 0.203: IC3.42 52.83,17.06 54,15.89 85.75,15.89 92.74,22.87 XIO.23
PWRIN
  Top 1.016: D1.A 18.31,2.81 17.04,4.08 17.04,4.2 15.39,5.85 15.27,5.85 13.49,7.63 12.4,7.63 X1.2
RD+
  Top 0.254: IC4.29 15.67,34.56 13.54,36.69 13.54,38.01 13.28,38.26 12.8,38.26 RN2.4
RD-
  Top 0.254: RN2.1 13.3,35.87 13.53,35.87 14,35.4 14,35.06 15,34.06 IC4.30
RESET  (via drill 0.41)
  Top 0.254: 46.83,19.46 46.56,19.19 44.22,19.19 43.71,19.7 | 28.82,17.88 28.18,17.88 27.33,17.03 27.33,15.89 RESET-EN.1
  Top 0.279: 46.83,19.46 IC3.30
  Top 0.305: POWER.3 33.05,7.89 v31.52,9.41 | 43.71,19.7 36.22,19.7 35.59,19.06 35.59,18.81 | 28.82,17.88 C7.2 | RESET-EN.1 RESET-EN.2 | RESET-EN.1 27.33,15.38 | 35.59,18.81 D3.A 34.36,16.32 C1.1 | RESET-EN.2 28.73,16.65 30.89,18.81 35.59,18.81 | RESET-EN.1 26.77,15.32 RN5.1 19.13,15.31 | RESET-EN.2 28.73,12.84 v28.09,12.2 | RESET.4 10.43,46.55 2.06,46.55 RESET.3 1.24,45.73 v1.24,43.14
  Top 0.406: v46.88,8.28 47.9,8.27 48.54,7.63 49.56,7.63 49.94,8.01 50.57,8.01 52.45,9.84 72.11,9.84 73.3,8.65 78.51,8.65 v78.64,8.78 | RESET.4 10.49,46.53
  Bottom 0.254: 63.78,25.29 64.29,24.78 64.29,17.79 66.7,15.38
  Bottom 0.305: v78.64,8.78 78.13,8.78 78,8.65 74.96,8.65 68.22,15.38 66.7,15.38 | 63.78,25.29 ICSP.5 | v46.88,8.28 45.75,9.28 31.65,9.28 v31.52,9.41 30.89,9.41 v28.09,12.2 27.99,12.1 1.35,12.1 0.69,12.76 0.69,42.58 v1.24,43.14
RESET2  (via drill 0.41)
  Top 0.254: IC4.24 16.54,38.94 16.54,39.13 | RN5.7 17.41,16.12 v16.54,15.25
  Top 0.305: ICSP1.5 15.01,47.51 | v16.54,15.25 16.61,15.32 | 16.54,39.13 16.54,39.51 v16.22,39.83 16.28,39.76 16.28,41.41 14.38,43.32 12.22,43.32 11.79,43.75 11.79,46.62 D2.A
  Top 0.61: D2.A 13.66,47.51 ICSP1.5
  Bottom 0.305: v16.54,15.25 16.79,15.25 16.79,21.22 19.46,23.76 19.46,29.1 20.6,30.24 23.27,30.24 23.52,30.49 23.52,33.14 18.17,38.49 17.68,38.49 16.47,39.7 v16.22,39.83
RXD1  (via drill 0.41)
  Top 0.203: IC3.45 54.36,20.36 54.34,20.4 54.34,18.36 55.32,17.36 71.98,17.36 v72.67,17.92
  Bottom 0.203: COMMUNICATION.3 81.31,42.68 74.19,35.57 74.19,19.57 v72.67,17.92
RXD2  (via drill 0.41)
  Top 0.203: IC3.12 41.06,28.86 v41.05,28.84
  Bottom 0.203: COMMUNICATION.5 76.23,49.29 75.72,48.78 74.07,48.78 73.69,48.4 68.3,48.4 67.41,49.29 64.62,49.29 63.73,48.4 63.65,48.4 60.73,45.48 58.7,45.48 56.67,47.51 51.33,47.51 50.06,46.24 44.48,46.24 43.71,45.48 43.71,38.98 40.31,35.57 40.31,30.44 41.02,29.73 41.02,28.87 v41.05,28.84
RXD3  (via drill 0.41)
  Top 0.203: COMMUNICATION.7 71.15,49.54 70.89,49.29 68.35,49.29 66.83,47.76 v66.83,47.38 | v55.78,29.73 55.78,29.48 56.92,28.33 58.83,28.33 IC3.63
  Bottom 0.203: v66.83,47.38 66.83,47 55.47,35.52 55.47,33.62 56.16,32.91 56.18,32.91 56.77,32.32 56.77,30.72 v55.78,29.73
RXL
  Top 0.254: 26.3,33.69 25.79,33.69 25.66,33.56 IC4.10
  Top 0.305: 26.3,33.69 RX.C
SCK2
  Top 0.254: ICSP1.3 19.46,48.65 22.25,48.65 23.52,47.38 23.52,39.26 22.89,38.62 22.89,37.86 23.52,37.22 23.52,36.46 23.12,36.06 IC4.15
SCL  (via drill 0.41)
  Top 0.203: IC3.43 53.33,17.32 54.25,16.4 74.7,16.4 75.08,16.78 v75.34,16.9 | v41.45,43.34 v44.96,43.34
  Top 0.254: 80.56,37.24 80.67,37.35 80.67,38.87
  Top 0.305: v81.43,39.13 80.92,39.13 80.67,38.87 | 80.56,37.24 RN1.2
  Bottom 0.203: COMMUNICATION.1 86.39,48.91 85.75,48.91 83.85,47 83.85,43.19 81.43,40.78 v81.43,39.13 80.04,39.13 75.21,34.3 75.21,17.03 v75.34,16.9 74.7,16.27 72.54,16.27 70.76,18.05 70.76,44.59 67.08,48.27 64.92,48.27 61.11,44.46 57.81,44.46 56.03,46.24 51.59,46.24 50.67,45.33 47.57,45.33 45.59,43.34 v44.96,43.34 | JP6.1 18.82,50.3 19.84,49.29 22.25,49.29 25.68,45.86 25.68,43.95 30.25,39.38 31.52,39.38 32.66,40.53 32.66,42.46 34.67,44.46 40.34,44.46 v41.45,43.34
SDA  (via drill 0.41)
  Top 0.203: v74.07,17.67 73.3,16.9 54.51,16.9 53.84,17.6 53.84,20.02 53.82,20.05 53.83,20.16 IC3.44 | v41.45,44.54 v44.96,44.54
  Top 0.305: v78.77,39 78.77,36.84 79.15,36.46 79.98,36.46 RN1.3
  Bottom 0.203: COMMUNICATION.2 83.85,49.54 82.58,48.27 82.58,42.81 v78.77,39 74.7,34.94 74.7,18.94 74.07,18.3 v74.07,17.67 74.07,17.03 73.81,16.78 72.67,16.78 71.27,18.17 71.27,44.72 67.21,48.78 64.8,48.78 60.99,44.97 58.32,44.97 56.41,46.88 51.46,46.88 50.37,45.78 46.89,45.78 45.64,44.54 v44.96,44.54 | JP6.2 21.49,50.81 26.19,46.11 26.19,44.21 30.51,39.89 31.27,39.89 32.16,40.78 32.16,42.68 34.52,45.05 40.94,45.05 v41.45,44.54
TXD1  (via drill 0.41)
  Top 0.203: IC3.46 54.83,20.27 54.84,20.27 54.84,18.75 55.65,17.92 70.76,17.92 v72.03,19.19
  Bottom 0.203: COMMUNICATION.4 78.77,42.56 73.69,37.48 73.69,20.08 72.67,19.19 v72.03,19.19
TXD2  (via drill 0.41)
  Top 0.203: IC3.13 41.83,28.36 41.43,27.95 39.9,27.95 39.78,28.08 v39.78,28.84
  Bottom 0.203: 39.78,29.22 v39.78,28.84 39.78,35.85 43.21,39.28 43.21,45.94 43.97,46.7 49.76,46.7 51.08,48.02 57.05,48.02 59.08,45.99 60.6,45.99 63.53,48.91 63.65,48.91 64.54,49.8 67.49,49.8 68.38,48.91 73.18,48.91 73.69,49.54 COMMUNICATION.6
TXD3  (via drill 0.41)
  Top 0.203: COMMUNICATION.8 68.35,50.81 67.72,50.18 67.72,49.8 v65.3,47.38 | IC3.64 58.68,28.86 58.57,28.84 57.68,28.84 57.3,29.22 57.3,30.37 v55.78,31.89
  Bottom 0.203: v65.3,47.38 65.3,46.24 54.99,35.9 54.99,32.68 v55.78,31.89
TXL
  Top 0.254: TX.C 26.82,36.84 24.04,34.06 IC4.11
UGND
  Top 0.254: IC4.28 16.23,35.06 15.67,35.62
  Top 0.406: 15.67,35.62 14.61,36.69 14.61,37.07 C10.2
  Top 0.813: X2.4 6.53,36.84 5.11,36.84 4.47,37.48 4.47,40.53 7.59,43.65 7.65,43.65 8.61,44.61 10.29,44.61 10.85,44.06 10.85,44.01 10.95,43.9 10.95,43.4 12.07,42.33 12.28,42.33 L1.1 13.94,41.52 14.55,40.91 14.55,37.33 C10.2
  Bottom 0.813: X2.4 6.55,36.55 GROUND.1
USBVCC
  Top 0.254: IC4.31 15.92,33.56 15.14,32.78 15.14,32.02 14.38,31.25
  Top 0.305: 14.38,31.25 13.23,31.25 C8.1
  Top 0.406: C8.1 12.98,31.51 12.34,32.14 10.82,32.14 10.19,31.51 10.19,28.59 11.58,27.19 11.58,25.9
  Top 0.61: 11.58,25.9 T1.1 6.99,24.73 F1.1
USHIELD  (via drill 0.41)
  Top 0.406: L1.2 10.89,41.36
  Top 0.813: X2.P$2 3.84,33.03 5.11,33.03 5.74,33.67 9.82,33.67 Z1.1 | v9.68,43.19 9.68,41.92 10.08,41.52 L1.2 11.09,41.31 Z2.1 | X2.P$1 4.64,44.92
  Bottom 0.813: v9.68,43.19 5.01,43.19 X2.P$1
  Bottom 1.27: X2.P$2 3.84,33.03 2.13,34.73 2.13,41.44 3.84,43.19 X2.P$1
VIN  (via drill 0.41)
  Top 0.203: 11.79,20.07 IC1.3
  Top 0.305: RN5.6 16.01,16.92 15.77,17.16
  Top 0.813: v24.03,7.38 22.62,7.38 PC1.+ 17.06,11.56 15.27,13.35 15.27,15.76 15.77,16.27 15.77,17.16 C2.1 12.86,20.07 11.79,20.07
  Top 1.016: D1.C 24.03,3.02 v24.03,7.38
  Bottom 1.27: v24.03,7.38 24.54,7.76 24.92,7.38 44.35,7.38 45.75,5.98 POWER.8
VUCAP
  Top 0.254: IC4.27 16.85,35.56 16.59,35.83
  Top 0.406: 16.59,35.83 16.28,36.13 16.28,37.17 C10.1
XT1
  Top 0.254: 17.83,29.35 R2.1 18.21,30.01 IC4.1
  Top 0.305: C14.1 16.15,26.3 Y2.2
  Top 0.406: C14.1 R2.1
XT2
  Top 0.254: IC4.2 18.71,29.96 R2.2 | C15.1 20.73,26.3 Y2.1
  Top 0.406: C15.1 R2.2
XTAL1
  Top 0.203: IC3.34 48.83,18.81 47.56,17.54 42.57,17.54
  Top 0.254: Y1.3 39.92,13.62 R1.1 40.92,13.73 41.68,14.49 41.68,16.9 42.32,17.54 42.57,17.54
XTAL2
  Top 0.203: 43.33,18.05 43.43,17.94 47.08,17.94 48.33,19.19 IC3.33
  Top 0.254: 37.86,15.62 Y1.1 37.98,15.62 38.09,15.51 R1.2 41.05,16.01 41.05,17.16 41.94,18.05 43.33,18.05
XVCC
  Top 0.61: F1.2 2.52,28.63 1.55,29.6 1.55,34.05 2.44,34.94 7.47,34.94 8.56,36.03 8.56,36.85 X2.1

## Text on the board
Bottom: Mega2560 Rev3E
tPlace: 9 | 8 | 7 | 6 | 5 | 4 | 3 | 2 | 1 | 0 | 22 | 14 | 15 | 16 | 17 | 18 | 19 | 20 | 21 | 13 | 12 | 11 | 10 | 24 | 26 | 28 | 30 | 31 | 32 | 33 | 34 | 35 | 36 | 37 | 38 | 39 | 40 | 41 | 42 | 43 | Arduino.org | 44 | 45 | 46 | 47 | TM | 48 | 49 | 50 | 51 | 52 | 53 | 0 | 1 | 2 | 3 | 4 | 5 | 6 | 7 | 8 | 9 | 10 | 11 | 12 | 13 | 14 | 15
tNames: SCL | SDA | 5V | GND | AREF | PWM | TX | RX | TX3 | RX3 | TX2 | RX2 | TX1 | RX1 | SDA | SCL | MADE IN | 1 | ITALY | DIGITAL | Arduino | MEGA 2560 | PC1 | PC2 | ANALOG IN | GND | IOREF | RESET | 3V3 | 5V | GND | VIN
bNames: MADE IN | designed by | ITALY | tinker it
ReferenceLC: L | ON | TX | RX
test-probe: SCL | SDA | AREF | GND3 | 13 | 12 | 11 | 10 | 9 | 8 | 7 | 6 | 5 | 4 | 3 | 2 | 1 | 0 | 14 | 15 | 16 | 17 | 18 | 19 | 20 | 21 | 5V_2 | 5V_3 | 22 | 23 | 24 | 25 | ISP2_6 | ISP2_4 | ISP2_2 | ISP2_1 | ISP2_3 | ISP2_5 | 26 | 27 | USB1_D+ | USB1_D- | 28 | 29 | 30 | 31 | USB1_GND | USB1_5V+ | 32 | 33 | 34 | 35 | ISP1_1 | ISP1_2 | 36 | 37 | ISP1_3 | ISP1_4 | 38 | 39 | ISP1_5 | ISP1_6 | 40 | 41 | 42 | 43 | 44 | 45 | 46 | 47 | 48 | 49 | 50 | 51 | DC_Vin- | DC_Vin+ | 52 | 53 | GND4 | GND5 | IOREF | RESET | 3V3 | 5V_1 | GND1 | GND2 | VIN | A0 | A1 | A2 | A3 | A4 | A5 | A6 | A7 | A8 | A9 | A10 | A11 | A12 | A13 | A14 | A15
